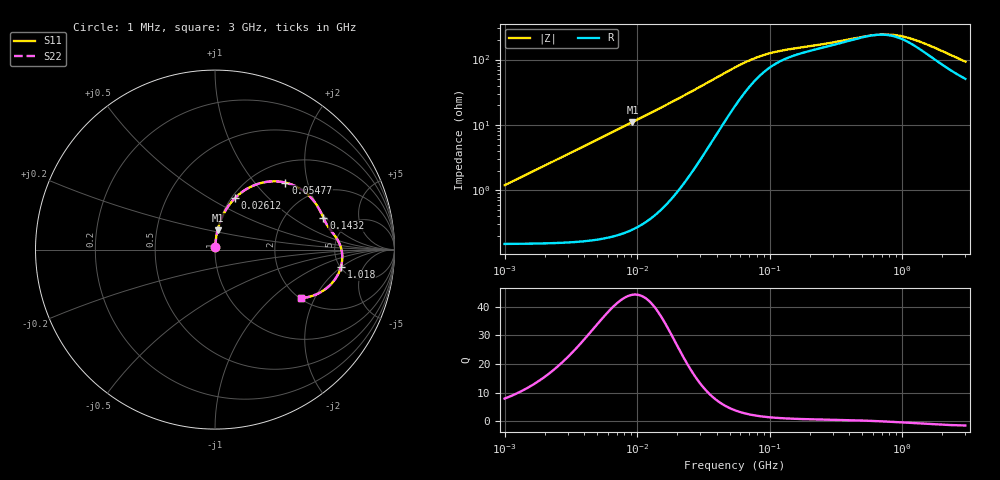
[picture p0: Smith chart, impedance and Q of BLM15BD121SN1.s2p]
! BLM15BD121SN1
# Hz S RI R 50
!Freq.(Hz) S11(Real) S11(Imag) S21(Real) S21(Imag) S12(Real) S12(Imag) S22(Real) S22(Imag)
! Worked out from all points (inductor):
!   401 points, 1 MHz to 3 GHz, reference 50 ohm
!   read as one part in series: L = 189 nH near 1.041 MHz
!   highest Q = 44.2 at 9.224 MHz (marker M1), where L = 191 nH
!   self-resonance near 632.2 MHz
!   S11 on the Smith chart (normalised r, x): 1 MHz: 1.00, +0.02; 26.12 MHz: 1.04, +0.66; 54.77 MHz: 1.39, +1.47; 143.2 MHz: 3.20, +1.88; 1.018 GHz: 5.05, -1.98; 3 GHz: 2.01, -1.56
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1000000  0.00165 0.0118  0.9984 -0.0118  0.9984 -0.0118  0.00165 0.0118
3823119  0.00369 0.0452  0.9963 -0.0452  0.9963 -0.0452  0.00369 0.0452
9223615  0.0144 0.1086  0.9856 -0.1086  0.9856 -0.1086  0.0144 0.1086
1.461624e7  0.0347 0.1704  0.9653 -0.1704  0.9653 -0.1704  0.0347 0.1704
2.013356e7  0.066 0.23  0.934 -0.23  0.934 -0.23  0.066 0.23
2.611722e7  0.1119 0.2873  0.8881 -0.2873  0.8881 -0.2873  0.1119 0.2873
3.190472e7  0.1661 0.3315  0.8339 -0.3315  0.8339 -0.3315  0.1661 0.3315
3.976269e7  0.248 0.3689  0.752 -0.3689  0.752 -0.3689  0.248 0.3689
4.666789e7  0.319 0.3802  0.681 -0.3802  0.681 -0.3802  0.319 0.3802
5.477226e7  0.392 0.3731  0.608 -0.3731  0.608 -0.3731  0.392 0.3731
6.826239e7  0.4795 0.3362  0.5205 -0.3362  0.5205 -0.3362  0.4795 0.3362
8.338914e7  0.5359 0.2882  0.4641 -0.2882  0.4641 -0.2882  0.5359 0.2882
1.060286e8  0.5764 0.232  0.4236 -0.232  0.4236 -0.232  0.5764 0.232
1.431579e8  0.6036 0.1776  0.3964 -0.1776  0.3964 -0.1776  0.6036 0.1776
2.094008e8  0.6277 0.1314  0.3723 -0.1314  0.3723 -0.1314  0.6277 0.1314
3.894533e8  0.6728 0.0702  0.3272 -0.0702  0.3272 -0.0702  0.6728 0.0702
5.696638e8  0.6994 0.0178  0.3006 -0.0178  0.3006 -0.0178  0.6994 0.0178
8.005644e8  0.7091 -0.0456  0.2909 0.0456  0.2909 0.0456  0.7091 -0.0456
1.017911e9  0.7014 -0.0976  0.2986 0.0976  0.2986 0.0976  0.7014 -0.0976
1.645649e9  0.6372 -0.2017  0.3628 0.2017  0.3628 0.2017  0.6372 -0.2017
2.266846e9  0.5586 -0.2519  0.4414 0.2519  0.4414 0.2519  0.5586 -0.2519
3e9  0.4764 -0.2705  0.5236 0.2705  0.5236 0.2705  0.4764 -0.2705
